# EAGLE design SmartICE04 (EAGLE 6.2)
AUTHOR: René König; REV: 2.01
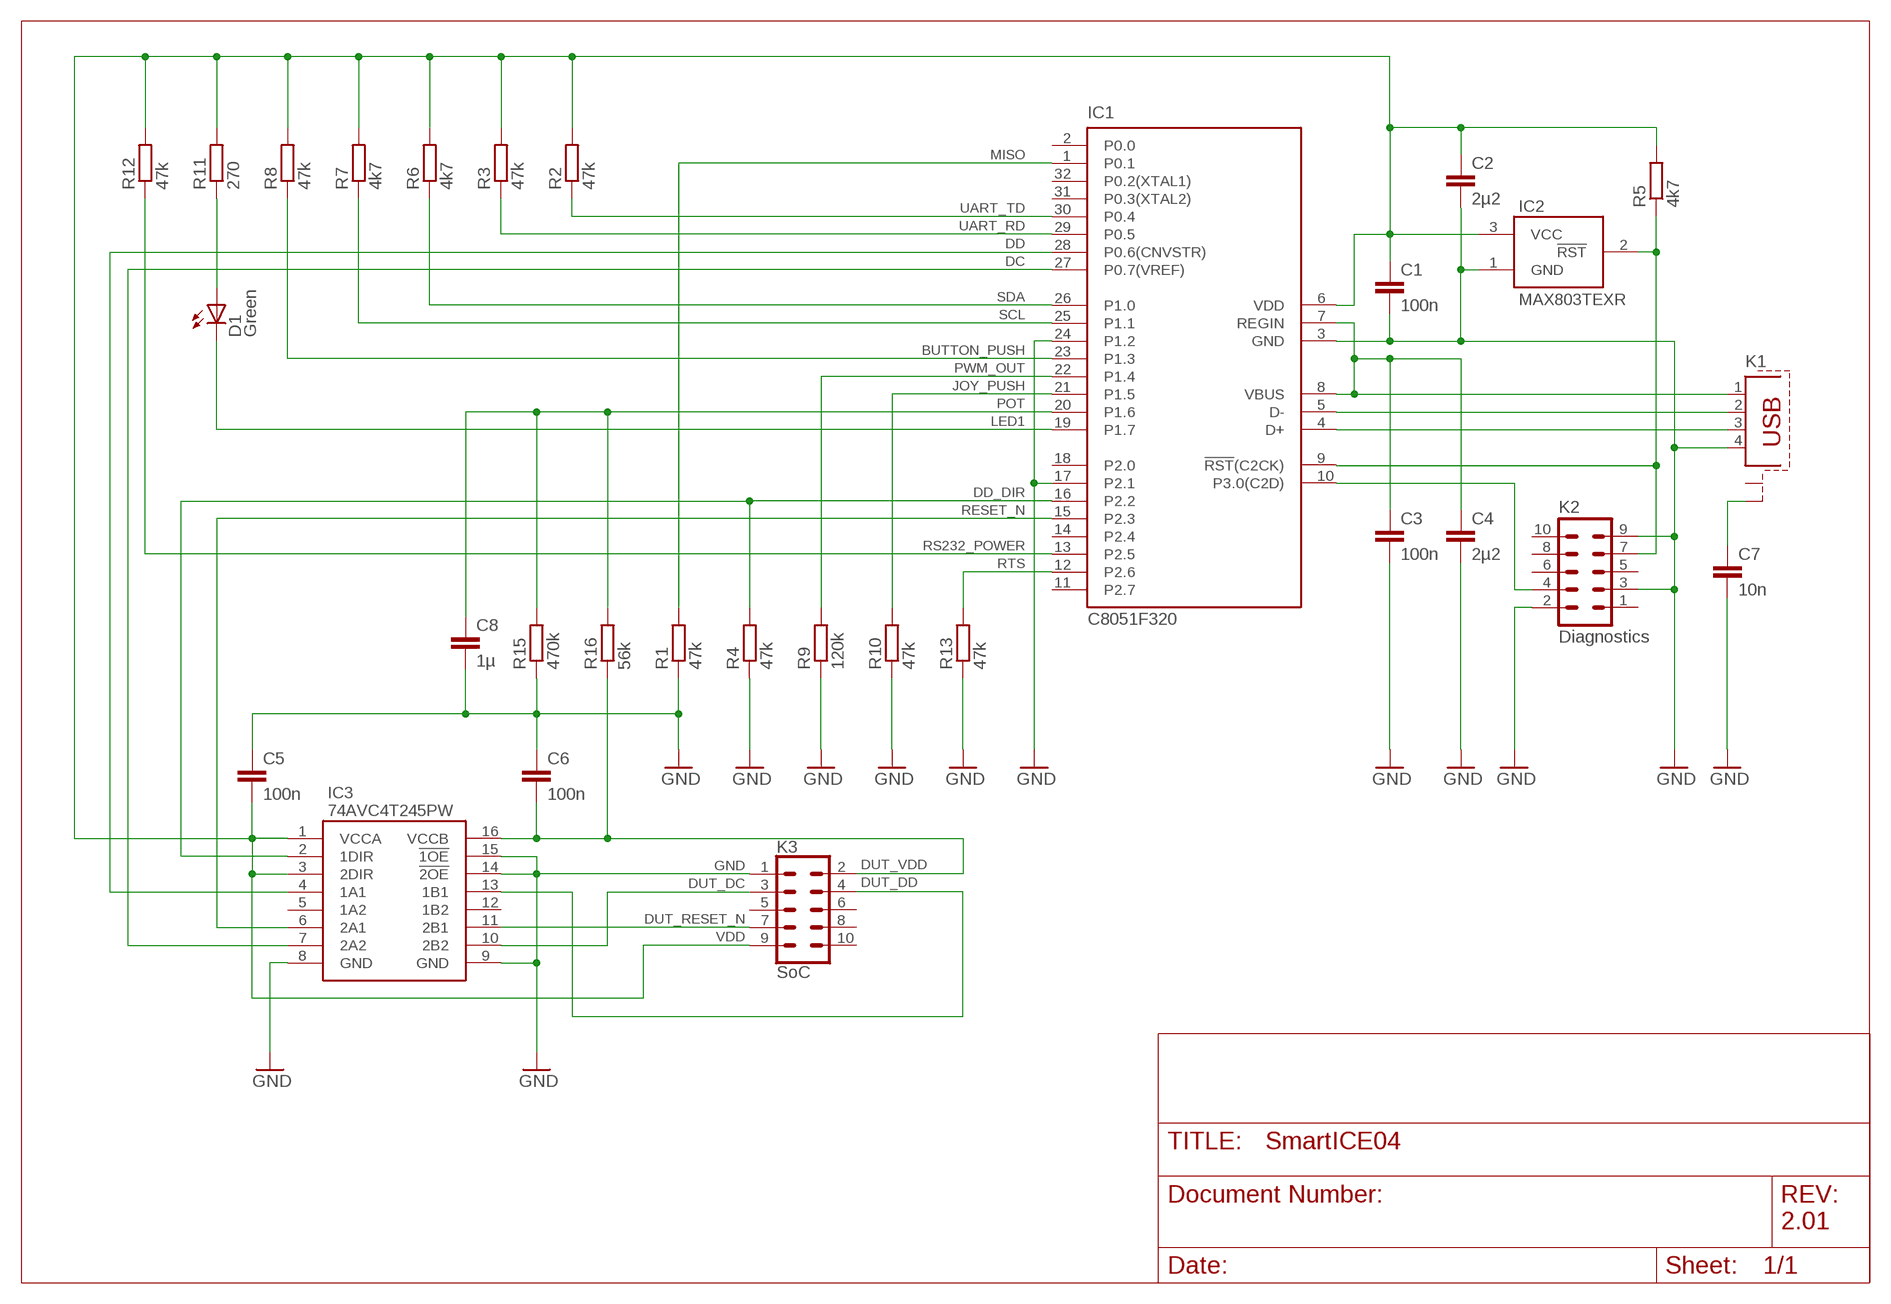
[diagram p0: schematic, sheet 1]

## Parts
C1  100n  C-EUC0805  [C0805]
C2  2µ2  C-EUC0805  [C0805]
C3  100n  C-EUC0805  [C0805]
C4  2µ2  C-EUC0805  [C0805]
C5  100n  C-EUC0805  [C0805]
C6  100n  C-EUC0805  [C0805]
C7  10n  C-EUC0805  [C0805]
C8  1µ  C-EUC0805  [C0805]
D1  Green  LED5MM  [LED5MM]
IC1  C8051F320  [TQFP32-08]
IC2  MAX803TEXR  [SC70-3L]
IC3  74AVC4T245PW  [R-PDSO-G16]
K1  PN61729-S  [PN61729-S]
K2  Diagnostics  ML10  [ML10]
K3  SoC  ML10L  [ML10L]
R1  47k  R-EU_R0805  [R0805]
R2  47k  R-EU_R0805  [R0805]
R3  47k  R-EU_R0805  [R0805]
R4  47k  R-EU_R0805  [R0805]
R5  4k7  R-EU_R0805  [R0805]
R6  4k7  R-EU_R0805  [R0805]
R7  4k7  R-EU_R0805  [R0805]
R8  47k  R-EU_R0805  [R0805]
R9  120k  R-EU_R0805  [R0805]
R10  47k  R-EU_R0805  [R0805]
R11  270  R-EU_R0805  [R0805]
R12  47k  R-EU_R0805  [R0805]
R13  47k  R-EU_R0805  [R0805]
R15  470k  R-EU_R0805  [R0805]
R16  56k  R-EU_R0805  [R0805]

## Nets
BUTTON_PUSH: IC1.23(P1.3) R8.1
C2D: IC1.10(P3.0(C2D)) K2.4
C2K: IC1.9(!RST!(C2CK)) IC2.2(!RST) K2.7 R5.1
D+: IC1.4(D+) K1.3
D-: IC1.5(D-) K1.2
DC: IC1.27(P0.7(VREF)) IC3.7(2A2)
DD: IC1.28(P0.6(CNVSTR)) IC3.4(1A1)
DD_DIR: IC1.16(P2.2) IC3.2(1DIR) R4.2
DUT_DC: IC3.10(2B2) K3.3
DUT_DD: IC3.13(1B1) K3.4
DUT_RESET_N: IC3.11(2B1) K3.7
DUT_VDD: C6.2 IC3.16(VCCB) K3.2 R16.1
GND: C1.2 C2.2 C3.2 C4.2 C5.1 C6.1 C7.2 C8.2 IC1.3(GND) IC1.17(P2.1) IC1.24(P1.2) IC2.1(GND) IC3.8(GND) IC3.9(GND) IC3.14(!2OE) IC3.15(!1OE) K1.4 K2.2 K2.3 K2.9 K3.1 R1.1 R4.1 R9.1 R10.1 R13.1 R15.1
JOY_PUSH [smsig]: IC1.21(P1.5) R10.2
LED1: D1.K(C) IC1.19(P1.7)
MISO: IC1.1(P0.1) R1.2
N$1: C7.1 K1.S2
N$8: D1.A R11.1
POT: C8.1 IC1.20(P1.6) R15.2 R16.2
PWM_OUT: IC1.22(P1.4) R9.2
RESET_N: IC1.15(P2.3) IC3.6(2A1)
RS232_POWER: IC1.13(P2.5) R12.1
RTS: IC1.12(P2.6) R13.2
SCL: IC1.25(P1.1) R7.1
SDA: IC1.26(P1.0) R6.1
UART_RD: IC1.29(P0.5) R3.1
UART_TD: IC1.30(P0.4) R2.1
VBUS: C3.1 C4.1 IC1.7(REGIN) IC1.8(VBUS) K1.1
VDD: C1.1 C2.1 C5.2 IC1.6(VDD) IC2.3(VCC) IC3.1(VCCA) IC3.3(2DIR) K3.9 R2.2 R3.2 R5.2 R6.2 R7.2 R8.2 R11.2 R12.2
Unconnected: IC1.2(P0.0) IC1.11(P2.7) IC1.14(P2.4) IC1.18(P2.0) IC1.31(P0.3(XTAL2)) IC1.32(P0.2(XTAL1)) IC3.5(1A2) IC3.12(1B2) K1.S1 K2.1 K2.5 K2.6 K2.8 K2.10 K3.5 K3.6 K3.8 K3.10

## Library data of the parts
C1-C8 = rcl:C-EU: CAPACITOR, European symbol
D1 = led:LED: LED
IC1 = TBKSiLabs:C8051F320: Full Speed USB, 16k ISP FLASH MCU; OC_FARNELL: 9685928; OC_NEWARK: 80K6691; OC_RS: 526-8857
IC2 = TBKMaxim:MAX803*: 3-Pin Microprocessor Reset Circuit; OC_FARNELL: 2085165; OC_RS: 732-7024
IC3 = TBKLogic:74AVC4T245: 4-BIT DUAL-SUPPLY BUS TRANSCEIVER WITH CONFIGURABLE VOLTAGE TRANSLATION AND 3-STATE OUTPUTS; OC_FARNELL: 1053499; OC_NEWARK: 33K5891; OC_RS: 663-1635
K1 = con-berg:PN61729-S: BERG USB connector; OC_FARNELL: unknown; OC_NEWARK: unknown
K2 K3 = con-harting-ml:ML10: HARTING; OC_FARNELL: unknown; OC_NEWARK: unknown
R1-R13 R15 R16 = rcl:R-EU_: RESISTOR, European symbol

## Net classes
0 default: width 0.3 mm
1 smsig: width 0.24 mm

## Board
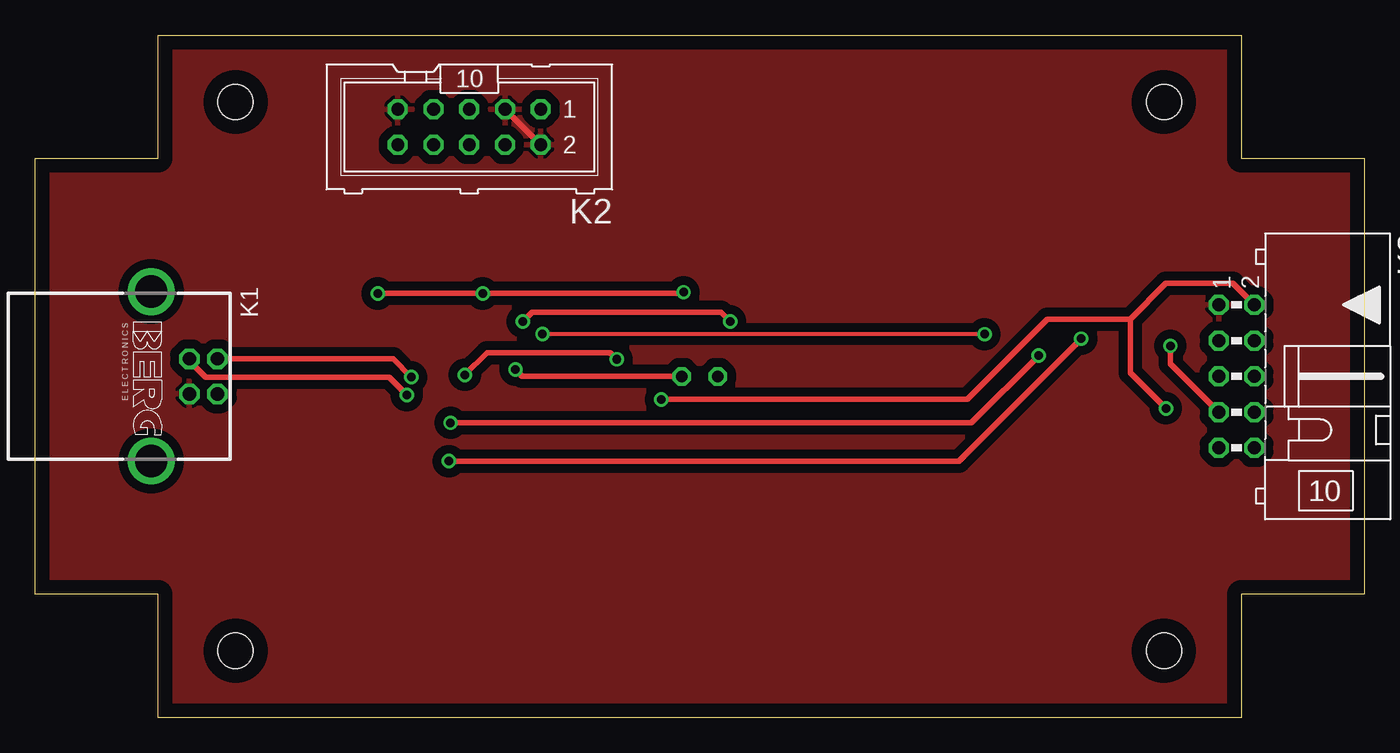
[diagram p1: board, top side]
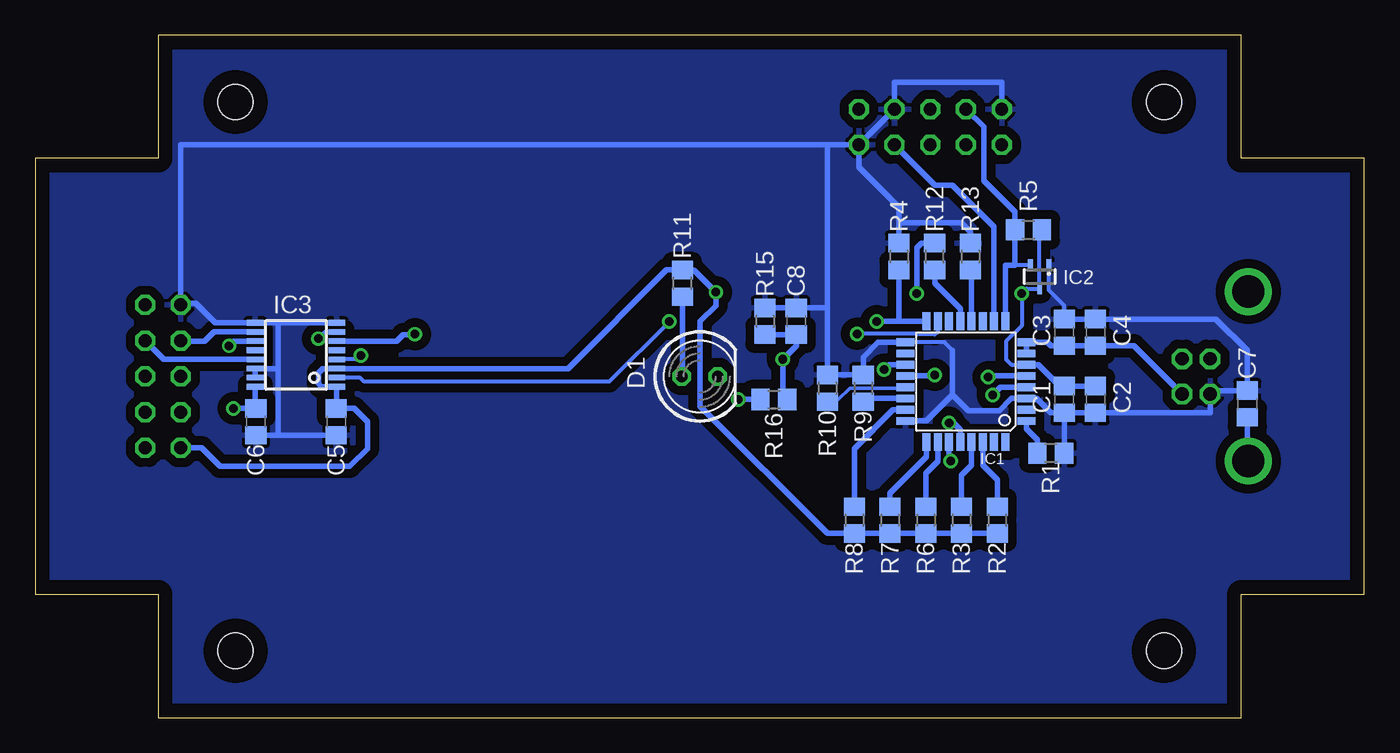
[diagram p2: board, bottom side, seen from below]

Size 94.5 x 48.5 mm. Coordinates in mm from the lower left corner, seen from the top.
Outline: 8.75,0 8.75,8.75 0,8.75 0,39.75 8.75,39.75 8.75,48.5 85.75,48.5 85.75,39.75 94.5,39.75 94.5,8.75 85.75,8.75 85.75,0 8.75,0
Copper layers (1*16): Top 0.035mm / dielectric 1.5mm / Bottom 0.035mm
Design rules "default": minimum track width 10mil, minimum drill 24mil, track to track 8mil, track to pad 6mil, pad to pad 8mil, via to via 8mil, smd to smd 8mil, copper to edge 40mil, drill to drill 8mil, minimum pad ring 10mil, minimum via ring 8mil, stop-mask expansion 4mil, vias tented up to drill 0mil, thermal gap 10mil
Holes 2.5 mm at 14.25,4.75 14.25,43.75 80.25,4.75 80.25,43.75

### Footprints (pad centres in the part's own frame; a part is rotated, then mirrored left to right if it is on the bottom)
C0805 = smd 1.3 x 1.5: 1 -0.95,0; 2 0.95,0
LED5MM = drill 0.813 octagon: A -1.27,0; K 1.27,0
TQFP32-08 = smd 1.27 x 0.559: 1 -4.293,2.8; 2 -4.293,2; 3 -4.293,1.2; 4 -4.293,0.4; 5 -4.293,-0.4; 6 -4.293,-1.2; 7 -4.293,-2; 8 -4.293,-2.8; 17 4.293,-2.8; 18 4.293,-2; 19 4.293,-1.2; 20 4.293,-0.4; 21 4.293,0.4; 22 4.293,1.2; 23 4.293,2; 24 4.293,2.8 | smd 0.559 x 1.27: 9 -2.8,-4.293; 10 -2,-4.293; 11 -1.2,-4.293; 12 -0.4,-4.293; 13 0.4,-4.293; 14 1.2,-4.293; 15 2,-4.293; 16 2.8,-4.293; 25 2.8,4.293; 26 2,4.293; 27 1.2,4.293; 28 0.4,4.293; 29 -0.4,4.293; 30 -1.2,4.293; 31 -2,4.293; 32 -2.8,4.293
SC70-3L = smd 0.35 x 0.8: 1 -0.65,-0.85; 2 0.65,-0.85; 3 0,0.85
R-PDSO-G16 = smd 0.4 x 1.2: 1 -2.275,-2.9; 2 -1.625,-2.9; 3 -0.975,-2.9; 4 -0.325,-2.9; 5 0.325,-2.9; 6 0.975,-2.9; 7 1.625,-2.9; 8 2.275,-2.9; 9 2.275,2.9; 10 1.625,2.9; 11 0.975,2.9; 12 0.325,2.9; 13 -0.325,2.9; 14 -0.975,2.9; 15 -1.625,2.9; 16 -2.275,2.9
PN61729-S = drill 0.95 octagon: 1 1.25,4.71; 2 -1.25,4.71; 3 -1.25,2.71; 4 1.25,2.71 | drill 2.3 pad 2.9: S1 -6.02,0; S2 6.02,0
ML10 = drill 0.914 octagon: 1 -5.08,-1.27; 2 -5.08,1.27; 3 -2.54,-1.27; 4 -2.54,1.27; 5 0,-1.27; 6 0,1.27; 7 2.54,-1.27; 8 2.54,1.27; 9 5.08,-1.27; 10 5.08,1.27
ML10L = drill 0.914 octagon: 1 -5.08,-1.27; 2 -5.08,1.27; 3 -2.54,-1.27; 4 -2.54,1.27; 5 0,-1.27; 6 0,1.27; 7 2.54,-1.27; 8 2.54,1.27; 9 5.08,-1.27; 10 5.08,1.27
R0805 = smd 1.3 x 1.5: 1 -0.95,0; 2 0.95,0

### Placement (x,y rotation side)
C1  21.34,22.61 270 bottom
C2  19.12,22.61 270 bottom
C3  21.34,27.37 90 bottom
C4  19.12,27.37 90 bottom
C5  73.09,21.02 90 bottom
C6  78.81,21.02 90 bottom
C7  8.32,22.29 90 bottom
C8  40.39,28.17 90 bottom
D1  47.25,24.25 0 bottom
IC1  28.32,23.88 180 bottom
IC2  23.09,31.34 180 bottom
IC3  75.95,25.79 90 bottom
K1  8.25,24.25 270 top
K2  30.86,41.98 180 top
K3  85.41,24.25 270 top
R1  22.29,18.8 180 bottom
R2  26.1,14.04 270 bottom
R3  28.64,14.04 270 bottom
R4  33.09,32.77 270 bottom
R5  23.88,34.67 0 bottom
R6  31.18,14.04 270 bottom
R7  33.72,14.04 270 bottom
R8  36.26,14.04 270 bottom
R9  35.63,23.4 270 bottom
R10  38.17,23.4 270 bottom
R11  48.49,30.86 90 bottom
R12  30.55,32.77 90 bottom
R13  28.01,32.77 270 bottom
R15  42.61,28.17 270 bottom
R16  41.98,22.61 0 bottom

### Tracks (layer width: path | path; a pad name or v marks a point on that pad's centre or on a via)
BUTTON_PUSH
  Bottom 0.406: IC1.23 33.5,21.88 36.26,19.12 R8.1
C2D
  Bottom 0.406: IC1.10 26.32,34.9 29.28,37.85 30.55,37.85 K2.4
C2K
  Bottom 0.3: 24.83,32.14 23.74,32.14 IC2.2
  Bottom 0.406: IC1.9 25.52,32.13 24.83,32.13 24.83,32.14 R5.1 24.83,35.95 27.05,38.17 27.05,41.98 K2.7
D+  (via drill 0.61)
  Top 0.406: K1.3 10.96,25.37 12.13,24.2 25.15,24.2 v26.42,22.93
  Bottom 0.406: v26.42,22.93 25.87,23.48 IC1.4
D-  (via drill 0.61)
  Top 0.406: K1.2 25.43,25.5 v26.74,24.2
  Bottom 0.406: IC1.5 26.66,24.28 v26.74,24.2
DC  (via drill 0.61)
  Top 0.406: v29.41,18.23 65.67,18.23 v74.37,26.93
  Bottom 0.3: IC3.7 73.89,27.41 v74.37,26.93
  Bottom 0.406: IC1.27 29.52,18.34 v29.41,18.23
DD  (via drill 0.61)
  Top 0.406: v29.53,20.95 66.57,20.95 v71.35,25.73
  Bottom 0.3: v71.35,25.73 71.61,25.47 IC3.4
  Bottom 0.406: IC1.28 28.73,20.47 29.28,21.02 29.46,21.02 v29.53,20.95
DD_DIR  (via drill 0.61)
  Top 0.406: v34.67,28.15 35.32,28.8 48.76,28.8 v49.41,28.15
  Bottom 0.3: v49.41,28.15 53.69,23.87 71.11,23.87 71.39,24.15 IC3.2
  Bottom 0.406: IC1.16 33.09,28.17 | 33.09,28.17 34.65,28.17 v34.67,28.15 | 33.09,28.17 R4.2
DUT_DC
  Bottom 0.406: IC3.10 81.79,27.41 82.46,26.74 84.09,26.74 K3.3
DUT_DD
  Bottom 0.406: IC3.13 85.35,25.46 K3.4
DUT_RESET_N  (via drill 0.61)
  Top 0.406: v80.71,26.42 80.71,25.14 K3.7
  Bottom 0.406: IC3.11 80.37,26.76 v80.71,26.42
DUT_VDD  (via drill 0.61)
  Top 0.406: K3.2 85.15,30.86 80.39,30.86 77.86,28.32 | v44.52,22.61 66.27,22.61 71.98,28.32 77.86,28.32 | v80.39,21.98 77.86,24.52 77.86,28.32
  Bottom 0.406: IC3.16 78.85,22.02 C6.2 v80.39,21.97 v80.39,21.98 | R16.1 v44.52,22.61
GND
  Top 0.406: K2.2 K2.3
  Bottom 0.3: IC2.1 22.44,30.37 21.34,29.28 C3.2 | IC1.17 29.86,26.68 29.28,26.1
  Bottom 0.406: C2.2 C1.2 | C2.2 18.8,21.66 | 18.8,21.66 C2.2 | R1.1 21.34,21.34 C1.2 | C1.2 22.29,21.66 23.32,22.68 IC1.3 25.08,22.68 25.94,21.82 28.17,21.82 29.28,22.93 | R10.1 R9.1 35.63,25.63 34.57,26.68 IC1.17 | R10.1 | C3.2 C4.2 10.54,28.32 8.32,26.1 C7.2 10.96,23.24 K1.4 10.96,22.93 10.96,21.66 18.8,21.66 | 77.22,20.07 C5.1 | 77.22,20.07 C6.1 | IC3.15 IC3.14 77.22,24.81 | 77.22,24.81 77.22,20.07 | 77.22,28.06 IC3.9 81.72,28.06 83.09,29.44 84.05,29.44 84.05,29.43 K3.1 84.14,40.71 38.17,40.71 | 77.22,28.06 77.22,24.81 | 77.22,28.06 IC3.8 | K2.9 25.79,45.15 33.41,45.15 K2.3 K2.2 | R13.1 28.01,34.52 28.64,35.15 33.09,35.15 | 33.09,35.15 R4.1 | 33.09,35.15 33.09,36.26 35.95,39.12 K2.2 | 38.17,40.71 K2.2 | R10.1 38.17,29.12 | 38.17,29.12 38.17,40.71 | IC1.24 31.12,21.08 29.28,22.93 | 29.28,22.93 29.28,26.1 | R15.1 C8.2 38.17,29.12
  pour Top (isolate 0.635): 8.75,0 8.75,8.75 0,8.75 0,39.75 8.75,39.75 8.75,48.5 85.75,48.5 85.75,39.75 94.5,39.75 94.5,8.75 85.75,8.75 85.75,0
  pour Bottom (isolate 0.635): 8.75,0 8.75,8.75 0,8.75 0,39.75 8.75,39.75 8.75,48.5 85.75,48.5 85.75,39.75 94.5,39.75 94.5,8.75 85.75,8.75 85.75,0
JOY_PUSH
  Bottom 0.26: IC1.21 32.69,23.4 36.58,23.4 37.37,22.61 38.17,22.61 R10.2
LED1  (via drill 0.61)
  Top 0.406: D1.K 34.63,24.25 v34.15,24.73
  Bottom 0.406: IC1.19 33.8,25.08 v34.15,24.73
MISO
  Bottom 0.406: IC1.1 24.03,20.54 23.25,19.75 R1.2
N$1
  Bottom 0.406: K1.S2 8.32,18.23 C7.1
N$8
  Bottom 0.406: R11.1 48.49,24.28 D1.A
POT  (via drill 0.61)
  Top 0.406: v30.55,24.36 32.13,25.94 40.87,25.94 v41.34,25.47
  Bottom 0.406: R15.2 C8.1 40.39,26.42 v41.34,25.47 41.34,22.93 R16.2 | IC1.20 30.62,24.28 v30.55,24.36
PWM_OUT
  Bottom 0.406: IC1.22 35.4,22.68 R9.2
RESET_N  (via drill 0.61)
  Top 0.3: v36.07,27.27 67.48,27.27 v67.5,27.25
  Bottom 0.3: v36.07,27.27 31.85,27.27 31.81,27.23 30.53,27.23 30.32,27.44 IC1.15
  Bottom 0.406: IC3.6 69.62,26.76 69.6,26.74 | 69.6,26.74 69.92,26.74 | 69.6,26.74 68.81,26.74 68.33,27.21 67.53,27.21 v67.5,27.25
RS232_POWER
  Bottom 0.406: IC1.13 28.73,29.04 30.55,30.86 R12.1
RTS
  Bottom 0.406: IC1.12 27.93,31.74 R13.2
SCL
  Bottom 0.406: IC1.25 31.12,18.54 33.72,15.94 R7.1 33.72,14.67
SDA
  Bottom 0.406: IC1.26 30.32,18.23 31.18,17.37 R6.1 31.18,14.67
UART_RD
  Bottom 0.406: IC1.29 27.93,17.93 28.64,17.21 R3.1
UART_TD
  Bottom 0.406: IC1.30 27.12,17.92 26.1,16.89 R2.1
VBUS
  Bottom 0.406: K1.1 16.38,26.42 C4.1 C3.1 22.29,26.42 22.55,26.68 IC1.8 24.03,26.74 24.04,26.74 IC1.7
VDD  (via drill 0.61)
  Top 0.406: v46.1,30.23 46.01,30.14 v31.82,30.14 v24.36,30.14
  Bottom 0.3: R5.2 23.09,34.52 IC2.3 24.01,30.49 v24.36,30.14 24.36,27.85 25.47,26.74 25.47,25.47 25.08,25.08 IC1.6
  Bottom 0.406: IC1.6 23.18,25.08 21.66,23.56 C1.1 C2.1 | 73.05,22.02 IC3.1 74.15,23.51 74.36,23.72 74.36,24.52 74.07,24.81 IC3.3 56.6,24.81 49.6,31.82 R11.2 | 73.05,22.02 C5.2 | K3.9 82.67,19.17 81.35,17.85 72.14,17.85 70.87,19.12 70.87,21.02 71.82,21.98 73.01,21.98 73.05,22.02 | R2.2 R3.2 R6.2 R7.2 | R7.2 34.04,13.09 R7.2 | R7.2 R8.2 38.17,13.09 47.22,22.13 47.22,28.17 46.1,29.28 46.1,30.05 46.01,30.14 v46.1,30.23 47.67,31.81 R11.2 | R12.2 31.5,33.72 31.82,33.41 v31.82,30.14 | R11.2 | R11.2 48.33,31.82 | R11.2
